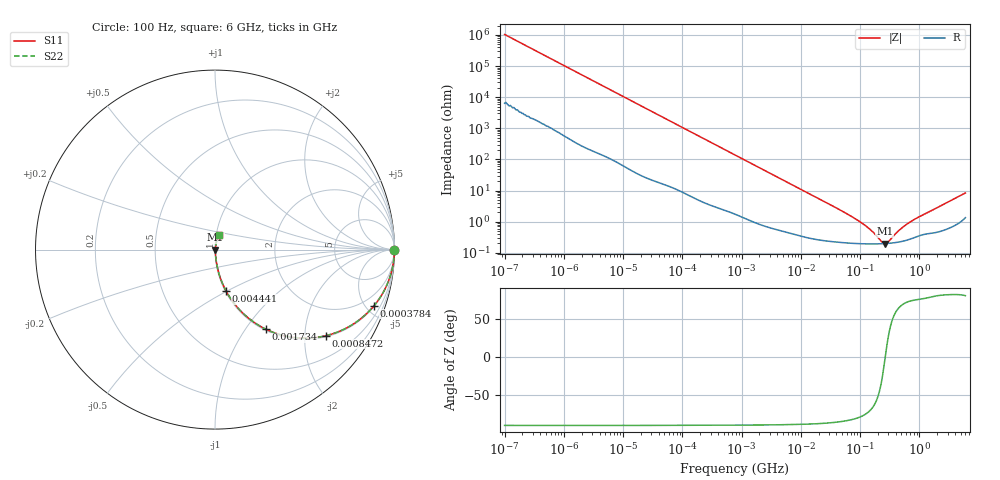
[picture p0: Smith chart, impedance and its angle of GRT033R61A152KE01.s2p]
!Murata Part Number: GRT033R61A152KE01
!These Parameters are Measured in Series Mode Connection
!Data Generated on Jun 19, 2026
!  o--ll--o
!Port1  Port2
!  o------o
!Operation Temp=25[degC], DC Bias Voltage=0[V]
!Freq. Start=100[Hz] Stop=6[GHz] 401[Steps]
# Hz S RI R 50
!Freq.(Hz) S11(Real) S11(Imag) S21(Real) S21(Imag) S12(Real) S12(Imag) S22(Real) S22(Imag)
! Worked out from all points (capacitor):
!   401 points, 100 Hz to 6 GHz, reference 50 ohm
!   read as one part in series: C = 1.53 nF near 109 Hz
!   lowest |Z| = 197 mohm at 261.2 MHz (marker M1)
!   series resonance near 266.1 MHz, so ESL is about 230 pH
!   S11 on the Smith chart (normalised r, x): 100 Hz: open; 378.4 kHz: 1.06, -5.67; 847.2 kHz: 1.03, -2.55; 1.734 MHz: 1.02, -1.25; 4.441 MHz: 1.01, -0.49; 6 GHz: 1.03, +0.16
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100  1 -9.61e-05  6e-07 9.61e-05  6e-07 9.61e-05  1 -9.61e-05
2008  1 -0.00191  1.35e-05 0.00191  1.35e-05 0.00191  1 -0.00191
40335  0.9983 -0.0379  0.0017 0.0379  0.0017 0.0379  0.9983 -0.0379
141303  0.9818 -0.1296  0.0182 0.1296  0.0182 0.1296  0.9818 -0.1296
378399  0.8871 -0.3115  0.1129 0.3115  0.1129 0.3115  0.8871 -0.3115
541393  0.7953 -0.3978  0.2047 0.3978  0.2047 0.3978  0.7953 -0.3978
774597  0.6581 -0.4682  0.3419 0.4682  0.3419 0.4682  0.6581 -0.4682
847162  0.6176 -0.4797  0.3824 0.4797  0.3824 0.4797  0.6176 -0.4797
1212075  0.4447 -0.4902  0.5553 0.4902  0.5553 0.4902  0.4447 -0.4902
1734173  0.2844 -0.444  0.7156 0.444  0.7156 0.444  0.2844 -0.444
2713602  0.1428 -0.3416  0.8572 0.3416  0.8572 0.3416  0.1428 -0.3416
4440638  0.0614 -0.2298  0.9386 0.2298  0.9386 0.2298  0.0614 -0.2298
1.555665e7  0.00776 -0.0702  0.9922 0.0702  0.9922 0.0702  0.00776 -0.0702
4.983056e7  0.00258 -0.0216  0.9974 0.0216  0.9974 0.0216  0.00258 -0.0216
9.753859e7  0.00205 -0.00995  0.998 0.00995  0.998 0.00995  0.00205 -0.00995
1.459435e8  0.00194 -0.00538  0.9981 0.00538  0.9981 0.00538  0.00194 -0.00538
2.283698e8  0.00194 -0.00129  0.9981 0.00129  0.9981 0.00129  0.00194 -0.00129
2.61201e8  0.00196 -0.000155  0.998 0.000155  0.998 0.000155  0.00196 -0.000155
3.124326e8  0.00201 0.00136  0.998 -0.00136  0.998 -0.00136  0.00201 0.00136
4.674818e8  0.00225 0.00498  0.9978 -0.00498  0.9978 -0.00498  0.00225 0.00498
7.31507e8  0.0029 0.00981  0.9971 -0.00981  0.9971 -0.00981  0.0029 0.00981
6e9  0.0197 0.0798  0.9803 -0.0798  0.9803 -0.0798  0.0197 0.0798
